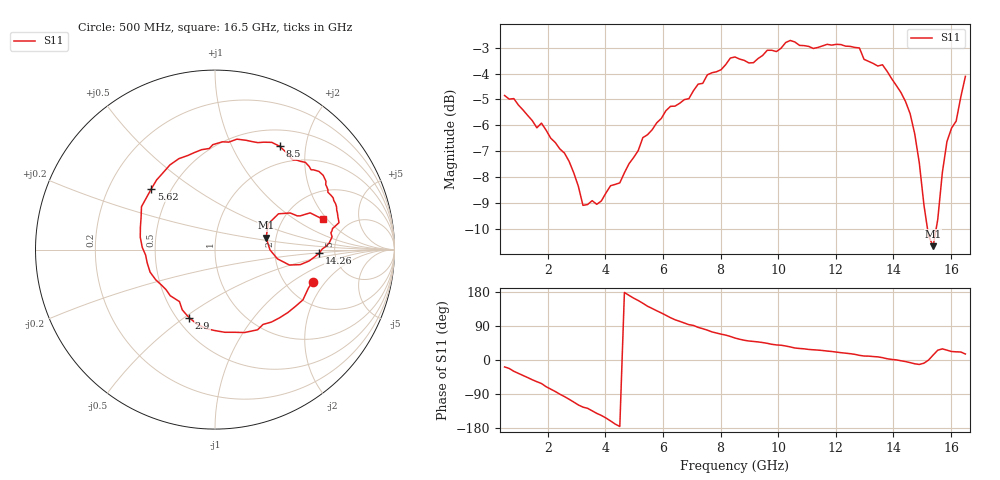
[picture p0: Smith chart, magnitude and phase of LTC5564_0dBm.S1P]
! LTC5564 S11 0 dBm source power.
! Reference plane is 1.1 mm from edge of QFN package.
! Measured 17-Jan 2013
# GHZ S DB R 50
!GHz	dB_S11	angS11
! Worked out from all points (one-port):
!   101 points, 500 MHz to 16.5 GHz, reference 50 ohm
!   lowest |S11| = -10.7 dB at 15.38 GHz (marker M1), VSWR 1.83, Z = 88.7 + j12.8 ohm
!   |S11| at or under -10 dB: 15.18 GHz to 15.49 GHz (303 MHz wide, 1.98 % of centre)
!   S11 on the Smith chart (normalised r, x): 500 MHz: 2.79, -1.49; 2.9 GHz: 0.57, -0.52; 5.62 GHz: 0.39, +0.35; 8.5 GHz: 0.73, +1.55; 14.26 GHz: 3.75, -0.23; 16.5 GHz: 3.23, +1.79
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0.5  -4.85 -18.3
1.14  -5.41 -40.8
1.78  -5.92 -62.0
2.58  -7.08 -96.6
2.9  -7.84 -111.0
3.22  -9.10 -124.4
4.02  -8.62 -153.1
4.5  -8.23 -175.5
5.3  -6.48 149.7
5.62  -6.18 136.1
6.26  -5.27 111.7
6.58  -5.15 102.0
7.54  -4.05 78.8
8.5  -3.36 58.0
8.98  -3.59 50.2
10.26  -2.80 37.0
10.58  -2.78 31.7
12.5  -2.95 16.7
12.98  -3.45 10.5
13.62  -3.66 6.2
14.26  -4.73 -2.0
14.58  -5.55 -6.9
14.9  -7.46 -11.7
15.22  -10.28 -0.2
15.38  -10.68 13.0
15.7  -7.83 29.4
16.34  -4.91 21.1
16.5  -4.11 15.8
